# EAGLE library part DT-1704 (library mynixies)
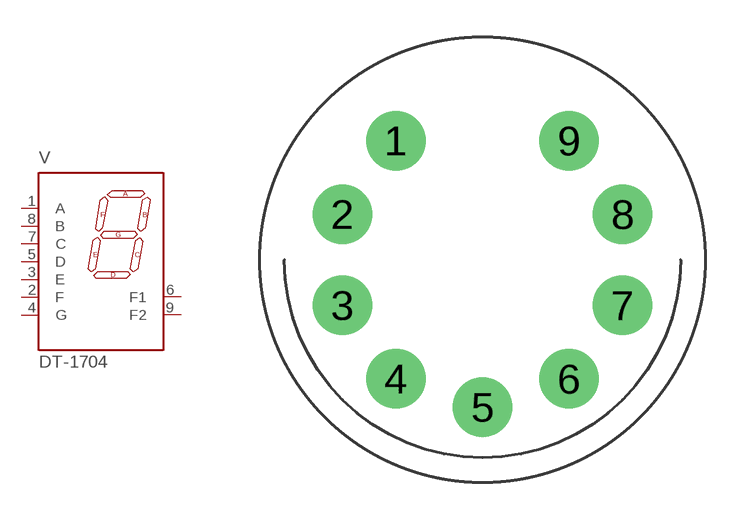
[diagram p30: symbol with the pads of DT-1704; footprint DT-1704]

Designator prefix V

## DT-1704  [DT-1704]
1  A  pas
2  F  pas
3  E  pas
4  G  pas
5  D  pas
6  F1  pas
7  C  pas
8  B  pas
9  F2  pas

## Footprint DT-1704 (pad centres in mm)
drill 1.6: 1 -3.497,4.814; 2 -5.659,1.839; 3 -5.659,-1.839; 4 -3.497,-4.814; 5 0,-5.95; 6 3.497,-4.814; 7 5.659,-1.839; 8 5.659,1.839; 9 3.497,4.814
